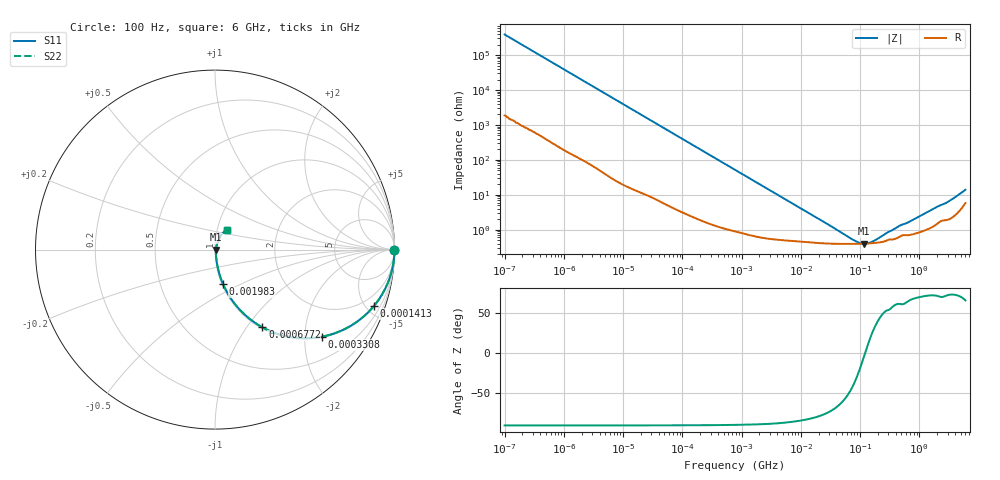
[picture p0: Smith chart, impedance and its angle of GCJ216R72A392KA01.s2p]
!Murata Part Number: GCJ216R72A392KA01
!These Parameters are Measured in Series Mode Connection
!Data Generated on Mar 13, 2026
!  o--ll--o
!Port1  Port2
!  o------o
!Operation Temp=25[degC], DC Bias Voltage=0[V]
!Freq. Start=100[Hz] Stop=6[GHz] 401[Steps]
# Hz S RI R 50
!Freq.(Hz) S11(Real) S11(Imag) S21(Real) S21(Imag) S12(Real) S12(Imag) S22(Real) S22(Imag)
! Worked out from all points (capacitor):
!   401 points, 100 Hz to 6 GHz, reference 50 ohm
!   read as one part in series: C = 4.08 nF near 109 Hz
!   lowest |Z| = 400 mohm at 116.7 MHz (marker M1)
!   series resonance near 121.6 MHz, so ESL is about 420 pH
!   S11 on the Smith chart (normalised r, x): 100 Hz: open; 141.3 kHz: 1.05, -5.65; 330.8 kHz: 1.03, -2.42; 677.2 kHz: 1.02, -1.19; 1.983 MHz: 1.01, -0.41; 6 GHz: 1.12, +0.25
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100  1 -0.000257  1.3e-06 0.000257  1.3e-06 0.000257  1 -0.000257
2008  0.9999 -0.00511  5.25e-05 0.00511  5.25e-05 0.00511  0.9999 -0.00511
12592  0.9988 -0.0318  0.00118 0.0318  0.00118 0.0318  0.9988 -0.0318
40335  0.9891 -0.1004  0.0109 0.1004  0.0109 0.1004  0.9891 -0.1004
82567  0.9574 -0.1982  0.0426 0.1982  0.0426 0.1982  0.9574 -0.1982
141303  0.8865 -0.3129  0.1135 0.3129  0.1135 0.3129  0.8865 -0.3129
211427  0.7793 -0.41  0.2207 0.41  0.2207 0.41  0.7793 -0.41
330837  0.5935 -0.4856  0.4065 0.4856  0.4065 0.4856  0.5935 -0.4856
473344  0.4192 -0.4869  0.5808 0.4869  0.5808 0.4869  0.4192 -0.4869
677235  0.2639 -0.4329  0.7361 0.4329  0.7361 0.4329  0.2639 -0.4329
774597  0.2165 -0.4034  0.7835 0.4034  0.7835 0.4034  0.2165 -0.4034
1212075  0.1051 -0.2958  0.8949 0.2958  0.8949 0.2958  0.1051 -0.2958
1983483  0.0453 -0.1937  0.9547 0.1937  0.9547 0.1937  0.0453 -0.1937
4856642  0.0119 -0.0823  0.9881 0.0823  0.9881 0.0823  0.0119 -0.0823
1.555665e7  0.00493 -0.0259  0.9951 0.0259  0.9951 0.0259  0.00493 -0.0259
7.797396e7  0.00392 -0.00313  0.9961 0.00313  0.9961 0.00313  0.00392 -0.00313
9.753859e7  0.00394 -0.00151  0.9961 0.00151  0.9961 0.00151  0.00394 -0.00151
1.166697e8  0.00397 -0.00028  0.996 0.00028  0.996 0.00028  0.00397 -0.00028
1.669249e8  0.00412 0.0022  0.9959 -0.0022  0.9959 -0.0022  0.00412 0.0022
3.124326e8  0.00524 0.00711  0.9948 -0.00711  0.9948 -0.00711  0.00524 0.00711
2.802721e9  0.0213 0.0528  0.9787 -0.0528  0.9787 -0.0528  0.0213 0.0528
6e9  0.068 0.1116  0.932 -0.1116  0.932 -0.1116  0.068 0.1116
